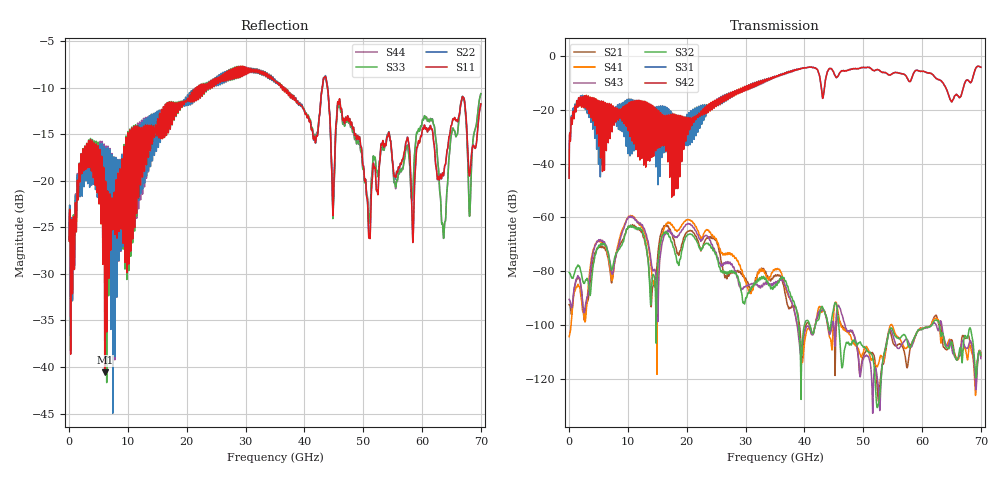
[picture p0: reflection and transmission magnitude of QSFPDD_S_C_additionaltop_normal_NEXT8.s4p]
! AWR Design Environment (8415) Thu Dec 20 13:49:17 2018
! Document = 'CHANNEL TEST'
! nPorts: 4, nXvals: 7001
# HZ S DB R 50
!Freq DBS11 AngS11 DBS12 AngS12 DBS13 AngS13 DBS14 AngS14
!	DBS21 AngS21 DBS22 AngS22 DBS23 AngS23 DBS24 AngS24
!	DBS31 AngS31 DBS32 AngS32 DBS33 AngS33 DBS34 AngS34
!	DBS41 AngS41 DBS42 AngS42 DBS43 AngS43 DBS44 AngS44
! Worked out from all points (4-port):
!   7000 points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, 10 MHz to 70 GHz, reference 50 ohm
!   strongest paths, dB at 10 MHz, 17.51 GHz, 35.01 GHz, 52.51 GHz, 70 GHz:
!     S42: -45.4, -28.7, -7.5, -5.0, -4.0
!     S31: -45.3, -23.9, -7.5, -5.0, -4.0
!     S32: -80.5, -69.3, -85.8, -130.1, -111.3
!     S43: -90.5, -65.9, -84.6, -121.6, -112.6
!     S41: -104.4, -62.6, -79.3, -115.0, -111.7
!     S21: -92.5, -66.1, -81.8, -127.4, -110.5
!   lowest |S11| = -40.5 dB at 6.06 GHz (marker M1), VSWR 1.02, Z = 49.4 + j0.738 ohm
!   |S11| at or under -10 dB: start of sweep to 21.77 GHz; 36.5 GHz to 43.04 GHz (6.538 GHz wide, 16.4 % of centre); 43.94 GHz to end of sweep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
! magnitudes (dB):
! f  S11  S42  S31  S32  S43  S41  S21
! 10 MHz  -26.5  -45.4  -45.3  -80.5  -90.5  -104.4  -92.5
! 1.64 GHz  -19.8  -15.4  -15.4  -78.2  -82.3  -85.6  -82.8
! 6.06 GHz  -40.5  -22.6  -18.8  -70.0  -69.3  -70.1  -71.3
! 20.33 GHz  -11.5  -22.8  -23.1  -66.4  -62.4  -60.8  -65.1
! 30.8 GHz  -8.1  -11.1  -11.4  -87.0  -84.9  -88.2  -86.8
! 63.65 GHz  -19.4  -10.2  -10.2  -104.5  -104.2  -104.5  -108.3
! 70 GHz  -11.8  -4.0  -4.0  -111.3  -112.6  -111.7  -110.5
